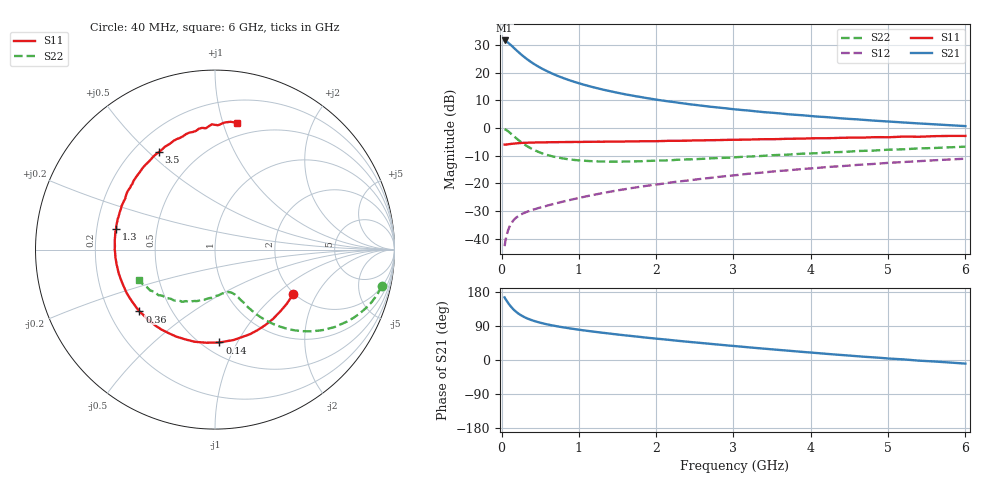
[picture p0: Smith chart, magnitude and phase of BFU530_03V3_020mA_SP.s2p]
! Filename:  P:\Prog\Test\Noise\ATS_data\Testdata_Net\03 Spar\BFU530_APG2013_40_A05_03p3V_020mA_SP_CM01_D.s2p
! Date/Time: Fri 26/Apr/2013 13:03:16
! BFU530_APG2013_40_A05_03p3V_1to25mA_SP_CM01_Bias7_R.s2p
! MDIF S-parameter v. bias file
! BFU530_APG2013_40_A05_03p3V_1to25mA_SP_CM01
! Date/time Wed Apr 24 18:17:07 2013
! VAR V_out= 3.3000
! VAR I_out= 20.0000
! VAR V_in= 0.8499
! VAR I_in= 0.2303
! Device data file deembeded for feedlines and parallel
! Original file: \03 Spar\BFU530_APG2013_40_A05_03p3V_020mA_SP_CM01_R.s2p
! Feed-files: PR047V01_250413_Feed1.s2p, PR047V01_250413_Feed2.s2p
! Parallel-file: PR047V01_250413_Par.s2p
# MHz S MA R 50
!  Freq-MHz  S11-mag  S11-arg  S21-mag  S21-arg  S12-mag  S12-arg  S22-mag  S22-arg
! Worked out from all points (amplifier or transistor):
!   98 points, 40 MHz to 6 GHz, reference 50 ohm
!   highest |S21| = 31.6 dB at 40 MHz (marker M1)
!   |S21| within 3 dB of that: start of sweep to 172 MHz
!   unconditionally stable (mu >= 1): 1.152 GHz to 3.431 GHz
!   at 300 MHz: K = 0.50, MSG = 28.1 dB, |S12| = -30.7 dB
!   at 1.6 GHz: K = 1.06, MAG = 15.7 dB, |S12| = -22.1 dB
!   at 6 GHz: K = 0.84, MSG = 5.9 dB, |S12| = -11.1 dB
!   S11 on the Smith chart (normalised r, x): 40 MHz: 1.96, -1.31; 140 MHz: 0.60, -0.85; 360 MHz: 0.33, -0.32; 1.3 GHz: 0.28, +0.10; 3.5 GHz: 0.30, +0.54; 6 GHz: 0.38, +1.11
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40  0.5016 -29.9  38.15 165.2  0.007292 79.4  0.9512 -12.4
50  0.5011 -37.2  37.73 161.2  0.008953 76.8  0.938 -15.4
80  0.5055 -56.5  35.12 152.2  0.01345 70.2  0.8815 -23.8
90  0.5075 -62.3  34.21 149.2  0.01473 68.3  0.8602 -26.2
120  0.5142 -78.3  31.6 141.2  0.01822 63.1  0.794 -32.9
140  0.518 -87.2  29.79 136.6  0.02013 60.4  0.7507 -36.6
180  0.5259 -102.4  26.38 128.7  0.0233 56.1  0.6707 -42.7
200  0.5271 -108.6  24.83 125.3  0.02455 54.5  0.6347 -45.2
240  0.5326 -119.3  22.15 119.6  0.02669 52.4  0.5725 -49.1
300  0.5385 -131.4  18.89 112.8  0.02933 50.6  0.4988 -53.5
360  0.5438 -140.7  16.35 107.5  0.03158 50.0  0.4437 -56.5
460  0.547 -151.8  13.25 100.7  0.03502 50.4  0.3785 -59.8
600  0.5506 -162.9  10.45 93.6  0.03972 52.0  0.3221 -62.5
800  0.5552 -173.7  7.966 86.1  0.04677 54.5  0.2804 -65.6
1050  0.5598 176.0  6.135 78.5  0.05615 56.9  0.2567 -69.3
1300  0.5632 168.1  4.981 72.1  0.06606 58.2  0.2476 -73.3
2050  0.5789 149.4  3.174 55.4  0.09676 58.2  0.257 -87.5
3100  0.6131 127.1  2.116 35.3  0.1434 54.0  0.2998 -107.9
3500  0.6257 119.9  1.883 28.1  0.1626 51.4  0.3214 -114.8
4100  0.6518 109.0  1.601 18.0  0.1902 47.0  0.3507 -126.2
5200  0.698 91.5  1.255 1.6  0.2422 37.8  0.4111 -145.1
6000  0.7167 80.1  1.08 -9.5  0.2779 30.0  0.4588 -158.1
